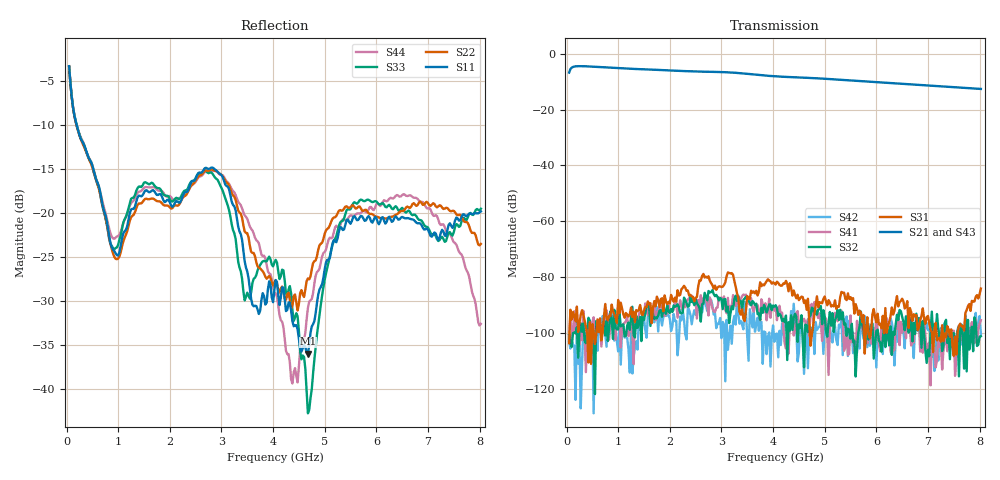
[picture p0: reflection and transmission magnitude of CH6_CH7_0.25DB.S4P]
!Agilent Technologies,E5071C,MY46316741,A.11.02
!Date: Mon Jun 01 10:33:03 2026
!Data & Calibration Information:
!1:CH6 INPUT 2:CH6 OUTPUT 3:CH7 INPUT 4:CH7 OUTPUT
!Freq	S11:SOLT4(ON)	S12:SOLT4(ON)	S13:SOLT4(ON)	S14:SOLT4(ON)
!	S21:SOLT4(ON)	S22:SOLT4(ON)	S23:SOLT4(ON)	S24:SOLT4(ON)
!	S31:SOLT4(ON)	S32:SOLT4(ON)	S33:SOLT4(ON)	S34:SOLT4(ON)
!	S41:SOLT4(ON)	S42:SOLT4(ON)	S43:SOLT4(ON)	S44:SOLT4(ON)
!PortZ  Port1:50+j0  Port2:50+j0  Port3:50+j0  Port4:50+j0
!Above PortZ is port z conversion or system Z0 setting when saving the data.
!When reading, reference impedance value at option line is always used.
# Hz S dB R 50
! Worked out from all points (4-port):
!   320 points, 50 MHz to 8.025 GHz, reference 50 ohm
!   strongest paths, dB at 50 MHz, 2.05 GHz, 4.05 GHz, 6.05 GHz, 8.025 GHz:
!     S21: -6.8, -6.0, -8.1, -10.2, -12.6
!     S43: -6.7, -6.0, -8.2, -10.3, -12.7
!     S31: -103.6, -87.8, -82.6, -96.9, -84.1
!     S32: -100.7, -92.4, -90.0, -102.7, -101.1
!     S41: -100.7, -91.8, -90.3, -103.9, -95.4
!     S42: -103.1, -97.6, -100.4, -104.6, -100.4
!   lowest |S11| = -36.0 dB at 4.675 GHz (marker M1), VSWR 1.03, Z = 48.7 - j0.905 ohm
!   |S11| at or under -10 dB: 195.1 MHz to end of sweep
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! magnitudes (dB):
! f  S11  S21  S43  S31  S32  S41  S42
! 50 MHz  -3.3  -6.8  -6.7  -103.6  -100.7  -100.7  -103.1
! 950 MHz  -24.6  -5.1  -5.1  -94.5  -98.0  -102.4  -98.8
! 2.8 GHz  -14.9  -6.5  -6.4  -82.1  -85.3  -88.6  -88.1
! 4.375 GHz  -32.3  -8.4  -8.5  -86.6  -98.9  -94.4  -97.1
! 4.675 GHz  -36.0  -8.6  -8.7  -87.7  -99.7  -95.0  -112.6
! 5.425 GHz  -20.8  -9.5  -9.5  -88.2  -101.0  -98.3  -94.1
! 8.025 GHz  -19.8  -12.6  -12.7  -84.1  -101.1  -95.4  -100.4
